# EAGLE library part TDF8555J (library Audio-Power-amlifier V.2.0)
The TDF8555J is one of a new generation of complementary quad Bridge-Tied Load (BTL) audio power amplifiers with full I2C-bus controlled diagnostics, multiple voltage regulator and two power switches intended for automotive applications. The TDF8555J can operate at a battery voltage as low as 6 V making this amplifier suitable for stop/start-car operation. The amplifier uses a complementary DMOS output stage in a Silicon-On-Insulator (SOI)-based BCD process. The DMOS output stage ensures a high power output signal with perfect sound quality. The SOI-based BCD process ensures a robust amplifier, where latch-up cannot occur, with good separation between the four independent channels with every component isolated and without substrate currents.
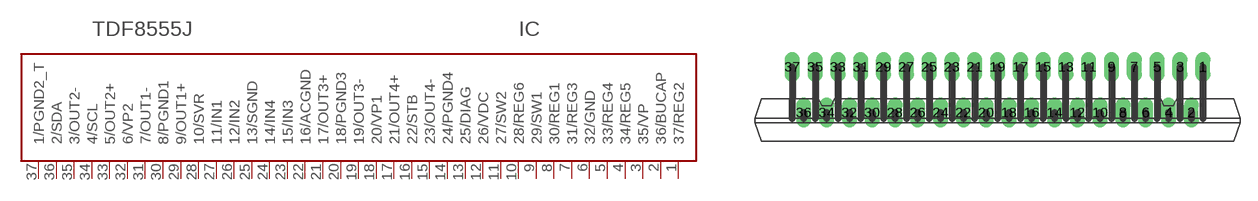
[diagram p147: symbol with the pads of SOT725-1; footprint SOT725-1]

Designator prefix IC

## TDF8555J  [SOT725-1]
1  37/REG2  out
2  36/BUCAP
3  35/VP  pwr
4  34/REG5  out
5  33/REG4  out
6  32/GND  pwr
7  31/REG3  out
8  30/REG1  out
9  29/SW1  out
10  28/REG6  out
11  27/SW2  out
12  26/VDC  pwr
13  25/DIAG  out
14  24/PGND4  pwr
15  23/OUT4-  out
16  22/STB  in
17  21/OUT4+  out
18  20/VP1  pwr
19  19/OUT3-  out
20  18/PGND3  pwr
21  17/OUT3+  out
22  16/ACGND  pwr
23  15/IN3  in
24  14/IN4  in
25  13/SGND  pwr
26  12/IN2  in
27  11/IN1  in
28  10/SVR
29  9/OUT1+  out
30  8/PGND1  pwr
31  7/OUT1-  out
32  6/VP2  pwr
33  5/OUT2+  out
34  4/SCL  in
35  3/OUT2-  out
36  2/SDA
37  1/PGND2_T  pwr

## Footprint SOT725-1 (pad centres in mm)
drill 0.8 long: 1 18,4; 2 17,0; 3 16,4; 4 15,0; 5 14,4; 6 13,0; 7 12,4; 8 11,0; 9 10,4; 10 9,0; 11 8,4; 12 7,0; 13 6,4; 14 5,0; 15 4,4; 16 3,0; 17 2,4; 18 1,0; 19 0,4; 20 -1,0; 21 -2,4; 22 -3,0; 23 -4,4; 24 -5,0; 25 -6,4; 26 -7,0; 27 -8,4; 28 -9,0; 29 -10,4; 30 -11,0; 31 -12,4; 32 -13,0; 33 -14,4; 34 -15,0; 35 -16,4; 36 -17,0; 37 -18,4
